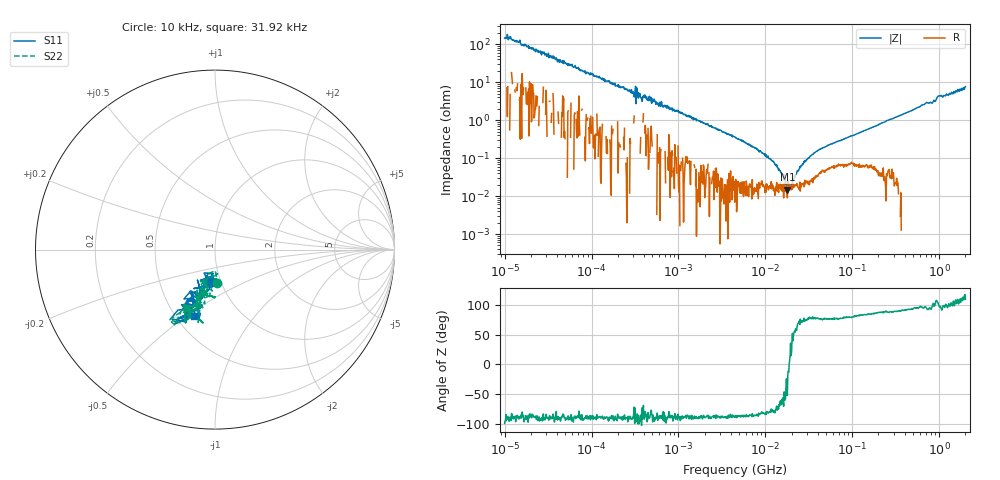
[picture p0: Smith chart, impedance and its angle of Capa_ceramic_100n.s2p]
#  HZ  S  MA  R  50.0
! Rohde & Schwarz ZVL
! 2 port VNA measurement of a 50 V X7R 100 nF ceramic capacitor (Murata GCM21BR71H104KA37L)
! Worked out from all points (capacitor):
!   1000 points, 10 kHz to 2 GHz, reference 50 ohm
!   read as one part in shunt: C = 97.5 nF near 10.63 kHz
!   lowest |Z| = 14.7 mohm at 17.9 MHz (marker M1)
!   series resonance near 18.78 MHz, so ESL is about 740 pH
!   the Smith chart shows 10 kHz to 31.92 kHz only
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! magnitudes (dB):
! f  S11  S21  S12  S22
! 10 kHz  -14.8  0.1  0.1  -14.5
! 11.3 kHz  -15.3  -0.1  -0.1  -15.0
! 42.8 kHz  -4.1  -1.9  -2.1  -4.3
! 76.94 kHz  -2.5  -4.3  -4.1  -2.5
! 199.6 kHz  -0.8  -10.5  -9.8  -0.4
! 337.5 kHz  -0.2  -13.8  -16.0  0.1
! 367.6 kHz  -1.3  -16.7  -14.1  0.2
! 592 kHz  -0.1  -20.4  -19.9  0.4
! 4.5 MHz  -0.1  -37.2  -37.2  -0.2
! 7.517 MHz  -0.1  -42.4  -42.5  -0.1
! 11.96 MHz  -0.1  -49.4  -49.1  0.0
! 14.36 MHz  -0.1  -53.6  -53.5  0.0
! 17.9 MHz  -0.1  -64.7  -62.2  -0.1
! 19.98 MHz  -0.1  -61.9  -61.8  0.0
! 24.59 MHz  0.0  -53.6  -53.2  0.1
! 34.62 MHz  -0.1  -46.2  -46.3  0.0
! 57.13 MHz  -0.1  -40.6  -40.5  0.0
! 263.1 MHz  -0.1  -27.9  -27.9  0.0
! 690.8 MHz  -0.3  -19.9  -20.2  -0.3
! 860.8 MHz  -0.5  -18.8  -19.1  -0.8
! 996.7 MHz  -0.7  -16.5  -16.6  -1.1
! 2 GHz  -0.6  -12.4  -13.6  -0.6
